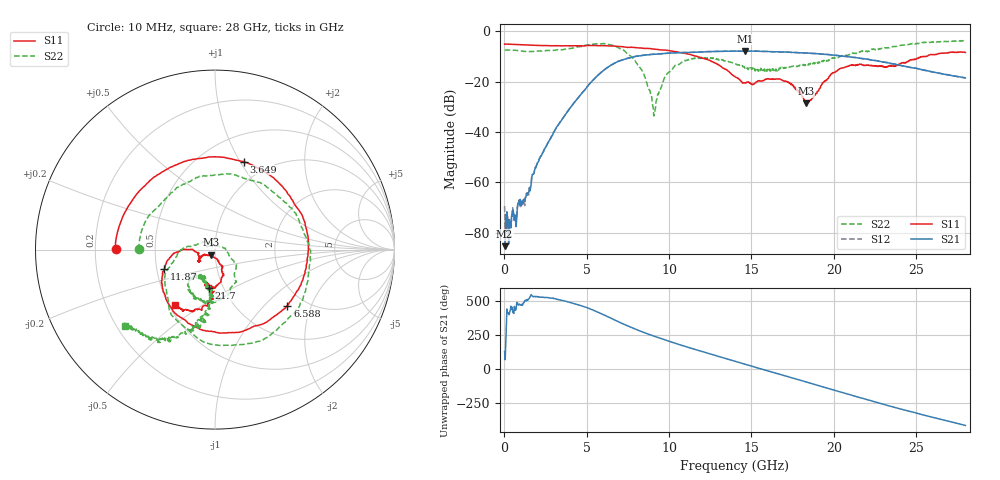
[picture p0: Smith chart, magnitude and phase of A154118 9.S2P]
!  2-Port S-parameters saved by WinCal
! VAR MeasName=S-Parameters (CALIBRATED_DATA) read from VNA (N5230A)
! VAR MeasDate=2015-9-10 14:35:05
! VAR NAME=A154118 9
! VAR FILENAME=A154118 9.S2P
! VAR DATE=2015-9-10 14:35:05
! VAR PHYS_PORTS=1,2
# Hz S DB R 50
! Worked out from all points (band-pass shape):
!   801 points, 10 MHz to 28 GHz, reference 50 ohm
!   highest |S21| = -7.85 dB at 14.6 GHz (marker M1); lowest = -85.3 dB at 10 MHz (marker M2)
!   |S21| within 3 dB of the highest: 7.427 GHz to 21.73 GHz (14.31 GHz wide, 98.1 % of centre)
!   lowest |S11| = -28.6 dB at 18.31 GHz (marker M3), VSWR 1.08, Z = 47.6 - j2.71 ohm
!   |S11| at or under -10 dB: 11.7 GHz to 25.48 GHz (13.78 GHz wide, 74.1 % of centre); 25.48668 GHz to 25.55638 GHz (69.71 MHz wide, 0.273 % of centre); 25.60111 GHz to 25.63285 GHz (31.73 MHz wide, 0.124 % of centre)
!   |S22| runs from -33.6 to -3.7 dB; largest |S21 - S12| = 0.0069
!   S11 on the Smith chart (normalised r, x): 10 MHz: 0.29, +0.00; 3.649 GHz: 0.78, +1.04; 6.588 GHz: 1.63, -1.38; 11.87 GHz: 0.55, -0.13; 21.7 GHz: 0.86, -0.39; 28 GHz: 0.54, -0.39
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1e7  -5.12 179.6  -85.30 130.4  -69.46 -24.9  -7.50 179.8
2.549125e8  -5.14 172.3  -84.50 56.3  -81.63 38.2  -7.45 172.1
6.747625e8  -5.26 160.5  -74.53 73.4  -74.62 83.2  -7.55 159.1
3.6487e9  -5.76 72.0  -33.56 142.1  -33.56 142.1  -7.17 60.8
4.698325e9  -5.84 33.6  -24.63 105.7  -24.59 105.5  -5.99 13.1
5.573012e9  -5.67 -0.1  -18.12 65.4  -18.10 65.5  -4.93 -33.8
6.58765e9  -5.85 -37.7  -13.04 9.0  -13.05 8.9  -5.55 -92.8
7.2874e9  -6.25 -59.7  -11.11 -30.2  -11.07 -30.1  -7.80 -129.2
8.302038e9  -6.63 -87.0  -9.71 -81.3  -9.64 -81.3  -15.14 177.0
9.071762e9  -7.09 -105.4  -9.14 -115.8  -9.07 -116.3  -33.60 92.9
9.351662e9  -7.30 -111.4  -9.07 -127.7  -8.97 -128.0  -25.02 6.5
1.03663e10  -8.09 -131.9  -8.60 -168.3  -8.56 -169.0  -13.58 -56.0
1.187076e10  -10.38 -158.9  -8.28 135.9  -8.25 135.3  -10.58 -97.5
1.4005e10  -18.01 179.3  -7.90 59.3  -7.91 58.9  -12.90 -130.1
1.459979e10  -20.46 -168.8  -7.85 38.2  -7.84 37.8  -14.62 -126.5
1.673402e10  -18.98 -145.8  -8.22 -36.8  -8.20 -37.7  -14.79 -108.8
1.830846e10  -28.56 -130.3  -8.62 -92.0  -8.61 -92.1  -13.63 -96.8
1.869332e10  -26.48 -89.4  -8.77 -105.5  -8.79 -105.9  -12.47 -96.0
1.995288e10  -16.51 -70.6  -9.50 -150.4  -9.45 -150.7  -10.75 -93.1
2.170225e10  -13.24 -98.4  -10.84 148.9  -10.83 148.1  -7.83 -100.1
2.334666e10  -13.84 -100.4  -12.57 92.2  -12.58 91.5  -6.56 -107.8
2.8e10  -8.42 -125.9  -18.51 -52.2  -18.55 -52.8  -3.66 -139.5
